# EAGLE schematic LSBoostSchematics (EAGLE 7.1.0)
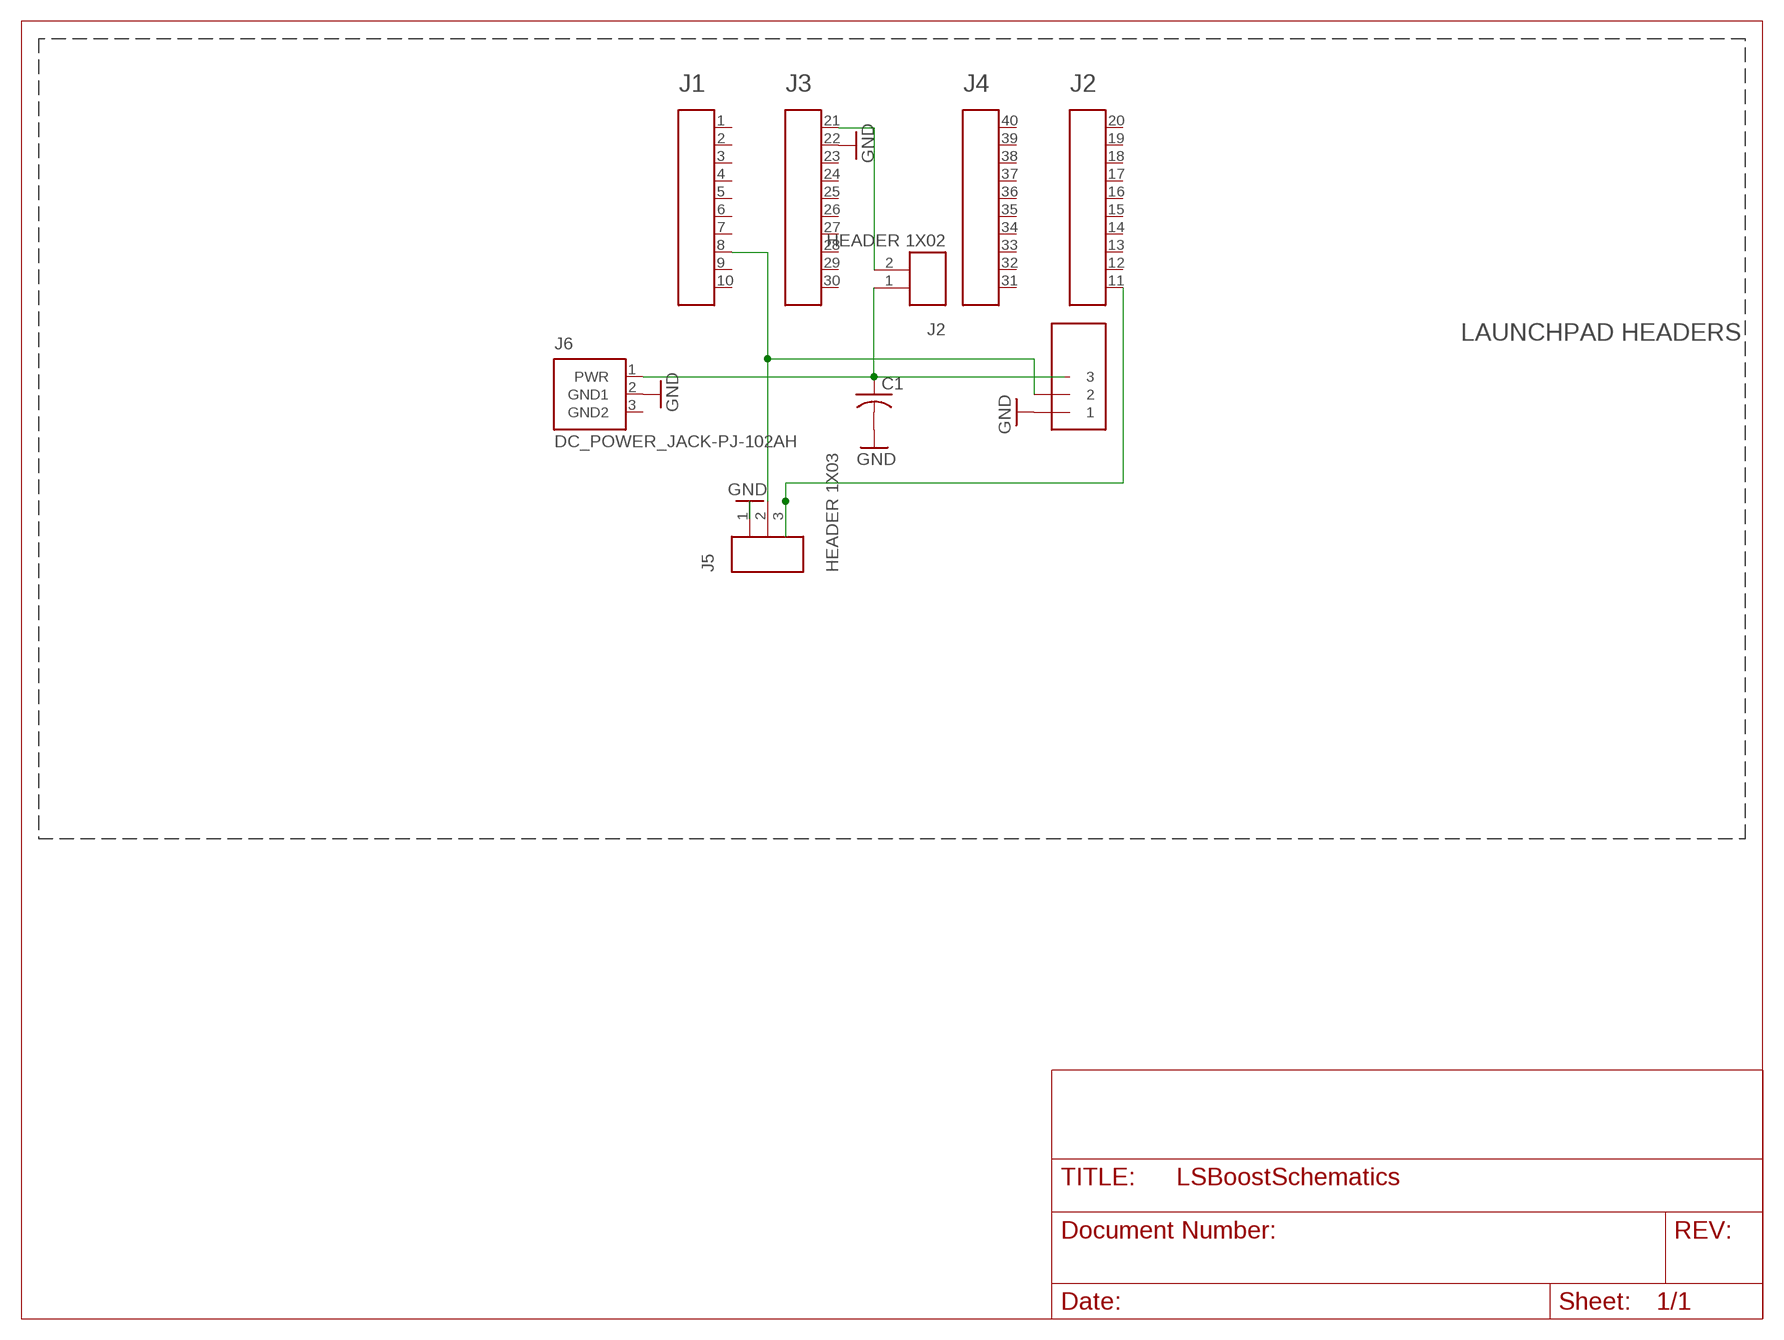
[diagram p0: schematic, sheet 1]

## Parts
A1  HEADER4X10-BOOSTERPACK  [4X10-BOOSTERPACK]
C1  C-US025-024X044  [C025-024X044]
J2  HEADER 1X02  HEADER1X02_100-TH  [1X02]
J5  HEADER 1X03  HEADER1X03_100-TH  [1X03]
J6  DC_POWER_JACK-PJ-102AH  [PJ-102AH]
J7  1X3  [1X3-3.5MM]

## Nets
GND: A1.21 A1.22 C1.2 J2.2 J5.1 J6.2(GND1) J7.1
N$2: A1.8 J5.2 J7.2
N$3: A1.11 J5.3
N$9: C1.1 J2.1 J6.1(PWR)
Unconnected: A1.1 A1.2 A1.3 A1.4 A1.5 A1.6 A1.7 A1.9 A1.10 A1.12 A1.13 A1.14 A1.15 A1.16 A1.17 A1.18 A1.19 A1.20 A1.23 A1.24 A1.25 A1.26 A1.27 A1.28 A1.29 A1.30 A1.31 A1.32 A1.33 A1.34 A1.35 A1.36 A1.37 A1.38 A1.39 A1.40 J7.3

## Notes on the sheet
- LAUNCHPAD HEADERS

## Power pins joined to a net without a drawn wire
GND2: J6.3(GND2)

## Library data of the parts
A1 = Public_BP_Library:HEADER4X10-BOOSTERPACK
C1 = adafruit:C-US: CAPACITOR, American symbol
J2 = EAGLE_BoosterPack_Library:HEADER1X02_; CCO: 258-0001290; DESCRIPTION: CONN HEADER .100 SINGL STR 2POS; MAN: SULLINS
J5 = EAGLE_BoosterPack_Library:HEADER1X03_; CCO: 258-0001299; DESCRIPTION: CONN HEADER .100 SINGL STR 3POS; MAN: SULLINS
J6 = connectors:DC_POWER_JACK: DC Power Jack
J7 = adafruit:1X3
